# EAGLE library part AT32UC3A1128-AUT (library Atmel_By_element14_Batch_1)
32-Bit Microcontroller
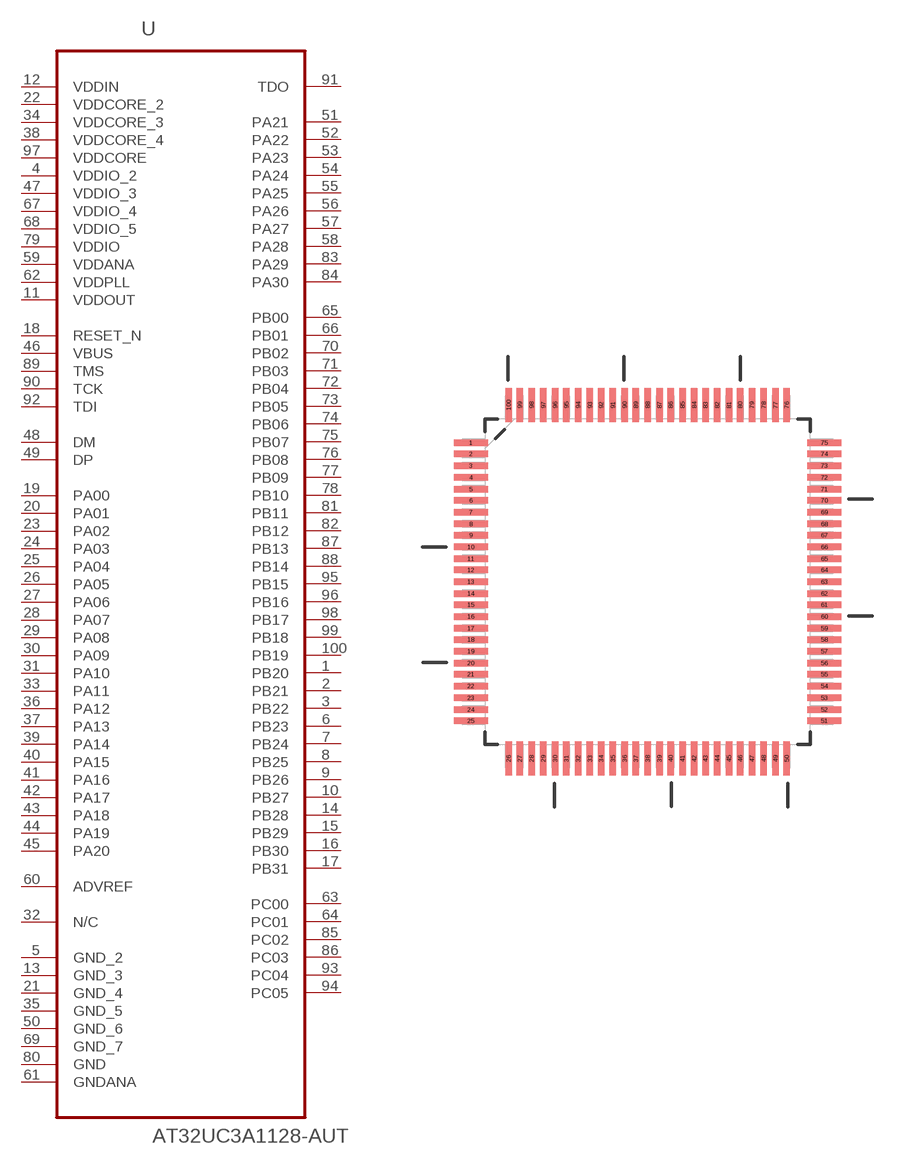
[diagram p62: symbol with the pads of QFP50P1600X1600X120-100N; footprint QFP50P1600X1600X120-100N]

Designator prefix U

## AT32UC3A1128-AUT (DESCRIPTION: 32-Bit Microcontroller; MPN: AT32UC3A1128-AUT; OC_FARNELL: 1841636; OC_NEWARK: 12T1370; PACKAGE: TQFP-100; SUPPLIER: Atmel Corporation)  [QFP50P1600X1600X120-100N]
1  PB20
2  PB21
3  PB22
4  VDDIO_2  pwr
5  GND_2  pas
6  PB23
7  PB24
8  PB25
9  PB26
10  PB27
11  VDDOUT  pwr
12  VDDIN  pwr
13  GND_3  pas
14  PB28
15  PB29
16  PB30
17  PB31
18  RESET_N  in
19  PA00
20  PA01
21  GND_4  pas
22  VDDCORE_2  pwr
23  PA02
24  PA03
25  PA04
26  PA05
27  PA06
28  PA07
29  PA08
30  PA09
31  PA10
32  N/C  nc
33  PA11
34  VDDCORE_3  pwr
35  GND_5  pas
36  PA12
37  PA13
38  VDDCORE_4  pwr
39  PA14
40  PA15
41  PA16
42  PA17
43  PA18
44  PA19
45  PA20
46  VBUS  in
47  VDDIO_3  pwr
48  DM  pas
49  DP  pas
50  GND_6  pas
51  PA21
52  PA22
53  PA23
54  PA24
55  PA25
56  PA26
57  PA27
58  PA28
59  VDDANA  pwr
60  ADVREF  pas
61  GNDANA  pas
62  VDDPLL  pwr
63  PC00
64  PC01
65  PB00
66  PB01
67  VDDIO_4  pwr
68  VDDIO_5  pwr
69  GND_7  pas
70  PB02
71  PB03
72  PB04
73  PB05
74  PB06
75  PB07
76  PB08
77  PB09
78  PB10
79  VDDIO  pwr
80  GND  pas
81  PB11
82  PB12
83  PA29
84  PA30
85  PC02
86  PC03
87  PB13
88  PB14
89  TMS  in
90  TCK  in
91  TDO  out
92  TDI  in
93  PC04
94  PC05
95  PB15
96  PB16
97  VDDCORE  pwr
98  PB17
99  PB18
100  PB19

## Footprint QFP50P1600X1600X120-100N (pad centres in mm)
smd 1.473 x 0.279: 1 -7.62,5.994; 2 -7.62,5.512; 3 -7.62,5.004; 4 -7.62,4.496; 5 -7.62,3.988; 6 -7.62,3.505; 7 -7.62,2.997; 8 -7.62,2.489; 9 -7.62,2.007; 10 -7.62,1.499; 11 -7.62,0.991; 12 -7.62,0.508; 13 -7.62,0; 14 -7.62,-0.508; 15 -7.62,-0.991; 16 -7.62,-1.499; 17 -7.62,-2.007; 18 -7.62,-2.489; 19 -7.62,-2.997; 20 -7.62,-3.505; 21 -7.62,-3.988; 22 -7.62,-4.496; 23 -7.62,-5.004; 24 -7.62,-5.512; 25 -7.62,-5.994; 51 7.62,-5.994; 52 7.62,-5.512; 53 7.62,-5.004; 54 7.62,-4.496; 55 7.62,-3.988; 56 7.62,-3.505; 57 7.62,-2.997; 58 7.62,-2.489; 59 7.62,-2.007; 60 7.62,-1.499; 61 7.62,-0.991; 62 7.62,-0.508; 63 7.62,0; 64 7.62,0.508; 65 7.62,0.991; 66 7.62,1.499; 67 7.62,2.007; 68 7.62,2.489; 69 7.62,2.997; 70 7.62,3.505; 71 7.62,3.988; 72 7.62,4.496; 73 7.62,5.004; 74 7.62,5.512; 75 7.62,5.994
smd 0.279 x 1.473: 26 -5.994,-7.62; 27 -5.512,-7.62; 28 -5.004,-7.62; 29 -4.496,-7.62; 30 -3.988,-7.62; 31 -3.505,-7.62; 32 -2.997,-7.62; 33 -2.489,-7.62; 34 -2.007,-7.62; 35 -1.499,-7.62; 36 -0.991,-7.62; 37 -0.508,-7.62; 38 0,-7.62; 39 0.508,-7.62; 40 0.991,-7.62; 41 1.499,-7.62; 42 2.007,-7.62; 43 2.489,-7.62; 44 2.997,-7.62; 45 3.505,-7.62; 46 3.988,-7.62; 47 4.496,-7.62; 48 5.004,-7.62; 49 5.512,-7.62; 50 5.994,-7.62; 76 5.994,7.62; 77 5.512,7.62; 78 5.004,7.62; 79 4.496,7.62; 80 3.988,7.62; 81 3.505,7.62; 82 2.997,7.62; 83 2.489,7.62; 84 2.007,7.62; 85 1.499,7.62; 86 0.991,7.62; 87 0.508,7.62; 88 0,7.62; 89 -0.508,7.62; 90 -0.991,7.62; 91 -1.499,7.62; 92 -2.007,7.62; 93 -2.489,7.62; 94 -2.997,7.62; 95 -3.505,7.62; 96 -3.988,7.62; 97 -4.496,7.62; 98 -5.004,7.62; 99 -5.512,7.62; 100 -5.994,7.62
